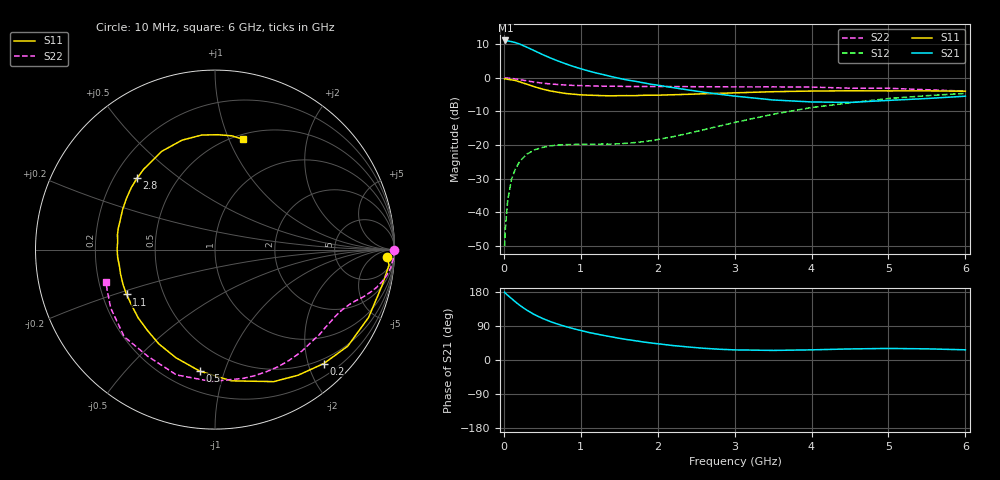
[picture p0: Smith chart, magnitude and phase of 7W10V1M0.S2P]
! Infineon Technologies  Discrete & RF Semiconductors
! BFS17W
! Si NPN RF Bipolar Junction Transistor in SOT323
! VCE = 10 V  IC = 1 mA
! Common Emitter S-Parameters:  August  1999
# GHz  S  MA  R  50
!  f  S11  S21  S12  S22
! GHz  MAG  ANG  MAG  ANG  MAG  ANG  MAG  ANG
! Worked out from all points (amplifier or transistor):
!   36 points, 10 MHz to 6 GHz, reference 50 ohm
!   highest |S21| = 11.2 dB at 20 MHz (marker M1)
!   |S21| within 3 dB of that: start of sweep to 391.8 MHz
!   unconditionally stable (mu >= 1): 1.085 GHz to 3.103 GHz; 4.099 GHz to end of sweep
!   at 250 MHz: K = 0.25, MSG = 16.8 dB, |S12| = -23.8 dB
!   at 1.4 GHz: K = 1.23, MAG = 7.2 dB, |S12| = -19.8 dB
!   at 6 GHz: K = 1.08, MAG = -2.1 dB, |S12| = -4.6 dB
!   S11 on the Smith chart (normalised r, x): 10 MHz: 25, -25; 200 MHz: 0.41, -2.28; 500 MHz: 0.33, -0.83; 1.1 GHz: 0.30, -0.22; 2.8 GHz: 0.29, +0.36; 6 GHz: 0.55, +1.12
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0.01  0.9601 -2.3  3.575 178.8  0.0031 84.8  0.9999 -0.1
0.02  0.9733 -5.1  3.617 176.4  0.0057 90.7  0.9961 -1.2
0.05  0.9523 -12.1  3.562 170.8  0.0149 84.6  0.9942 -3.1
0.1  0.9354 -23.8  3.474 162.2  0.031 76.7  0.9834 -6.1
0.15  0.9147 -36.0  3.358 153.4  0.0436 69.4  0.9658 -8.8
0.2  0.8778 -46.3  3.22 145.5  0.0553 64.8  0.9456 -11.1
0.25  0.8392 -56.5  3.039 138.1  0.0642 59.2  0.9239 -13.2
0.3  0.8051 -66.0  2.865 131.4  0.073 54.9  0.9038 -14.9
0.4  0.7368 -82.9  2.535 119.5  0.0848 47.7  0.8657 -17.8
0.5  0.682 -97.2  2.238 110.0  0.0917 42.8  0.8363 -19.8
0.6  0.6408 -109.8  1.995 101.7  0.0969 39.8  0.8137 -21.7
0.7  0.6117 -120.7  1.795 94.7  0.0996 37.7  0.7974 -23.6
0.9  0.5721 -138.6  1.487 82.9  0.1017 35.5  0.7735 -27.2
1.1  0.5527 -153.1  1.27 72.9  0.1032 36.6  0.7613 -31.1
1.6  0.5453 179.6  0.932 54.0  0.106 46.4  0.7455 -41.8
2.2  0.5609 156.7  0.716 38.1  0.1332 63.4  0.7427 -56.4
2.8  0.5887 137.6  0.571 28.4  0.1914 71.6  0.7362 -72.3
3.5  0.6229 118.4  0.469 25.3  0.2876 70.4  0.7353 -91.5
4  0.6367 106.8  0.438 26.8  0.3614 65.1  0.7302 -107.1
4.5  0.6426 96.6  0.431 29.2  0.4254 58.3  0.7026 -122.1
5.5  0.6409 81.6  0.493 29.4  0.5431 44.0  0.6662 -150.7
6  0.6341 76.0  0.534 26.9  0.5886 37.2  0.6355 -163.5
